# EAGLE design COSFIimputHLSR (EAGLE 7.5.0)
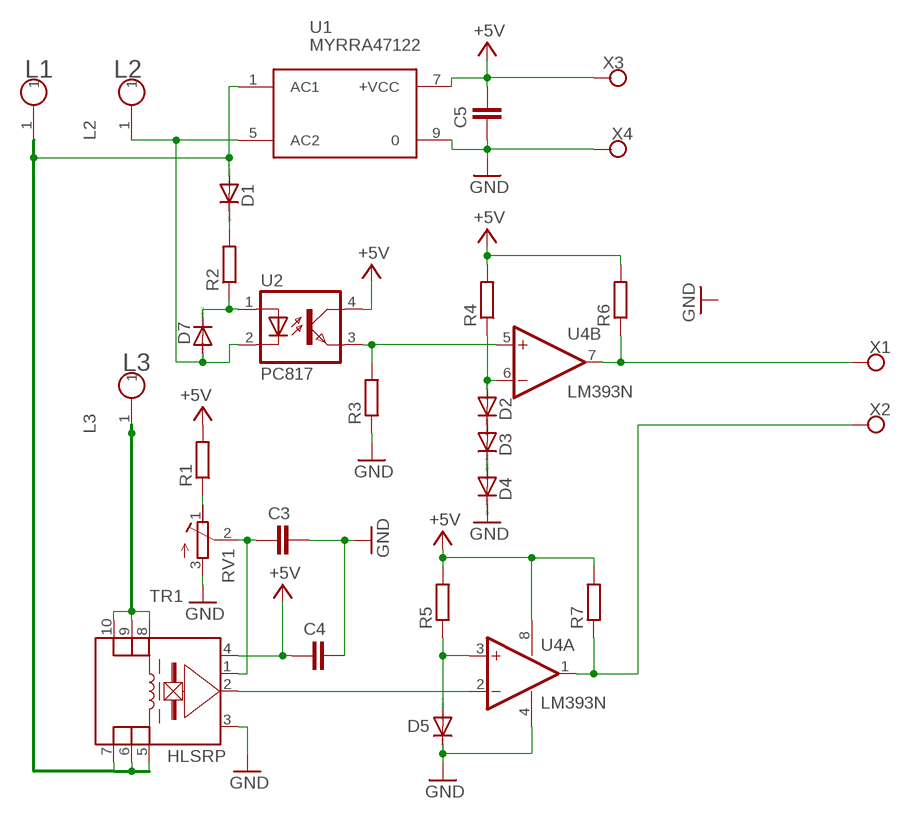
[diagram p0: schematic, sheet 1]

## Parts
C3  C-EUC1206  [C1206]
C4  C-EUC1206  [C1206]
C5  C-EUC1206  [C1206]
D1  1N4004  [DO41-10]
D2  1N4148DO35-7  [DO35-7]
D3  1N4148DO35-7  [DO35-7]
D4  1N4148DO35-7  [DO35-7]
D5  1N4148DO35-7  [DO35-7]
D7  1N4004  [DO41-10]
L1  CONNHOLE  [CONNHOLE4]
L2  CONNHOLE  [CONNHOLE4]
L3  CONNHOLE  [CONNHOLE4]
R1  R-EU_0207/10  [0207/10]
R2  R-EU_0617/22  [0617/22]
R3  R-EU_0204/7  [0204/7]
R4  R-EU_0204/7  [0204/7]
R5  R-EU_0204/7  [0204/7]
R6  R-EU_0204/7  [0204/7]
R7  R-EU_0204/7  [0204/7]
RV1  R-TRIMM-3386-F  [R-TRIMM-3386F]
TR1  HLSRP  [HLRSXPSP]
U1  MYRRA47122  [MYRRA47122]
U2  PC817  [DIL04]
U4  LM393N  [DIL08]
X1  CONNWIRE  [CONNWIRE]
X2  CONNWIRE  [CONNWIRE]
X3  CONNWIRE  [CONNWIRE]
X4  CONNWIRE  [CONNWIRE]

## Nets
+5V: C4.1 C5.2 R1.2 R4.2 R5.2 R6.2 R7.2 TR1.4(V+) U1.7(+VCC) U2.4(COL) U4.8(P:V+) X3.P$1
GND: C3.2 C4.2 C5.1 D4.C D5.C R3.1 RV1.3(E) TR1.3 U1.9 U4.4(P:V-) X4.P$1
N$1: TR1.2 U4.2(A:-IN)
N$2: D5.A R5.1 U4.3(A:+IN)
N$3: D7.C R2.1 U2.1(A)
N$4: D2.C D3.A
N$5: D7.A L2.1 U1.5(AC2) U2.2(C)
N$6: D1.A L1.1 TR1.5(4I-) TR1.6(5I-) TR1.7(6I-) U1.1(AC1)
N$7: C3.1 RV1.2(S) TR1.1
N$8: D3.C D4.A
N$9: R1.1 RV1.1(A)
N$10: D1.C R2.2
N$13: R3.2 U2.3(EMIT) U4.5(B:+IN)
N$16: D2.A R4.1 U4.6(B:-IN)
N$17: R7.1 U4.1(A:OUT) X2.P$1
N$18: R6.1 U4.7(B:OUT) X1.P$1
N$19: L3.1 TR1.8(1I+) TR1.9(2I+) TR1.10(3I+)

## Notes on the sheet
- L1 | L2
- L3

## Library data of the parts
C3-C5 = rcl:C-EU: CAPACITOR, European symbol
D1 D7 = diode:1N4004: DIODE
D2-D5 = diode:1N4148: DIODE
L1-L3 = connholes:CONNHOLE
R1-R7 = rcl:R-EU_: RESISTOR, European symbol
RV1 = rcl:R-TRIMM-3386-F
TR1 = lem:HLSRP
U1 = acdc:MYRRA47122: AC-DC CONVERTER 5V 550mA
U2 = optocoupler:PC817: SHARP OPTO COUPLER; MPN: PC817X4J000F; OC_FARNELL: 9707727; OC_NEWARK: 97K7059
U4 = linear:LM393: COMPARATOR
X1-X4 = connholes:CONNWIRE

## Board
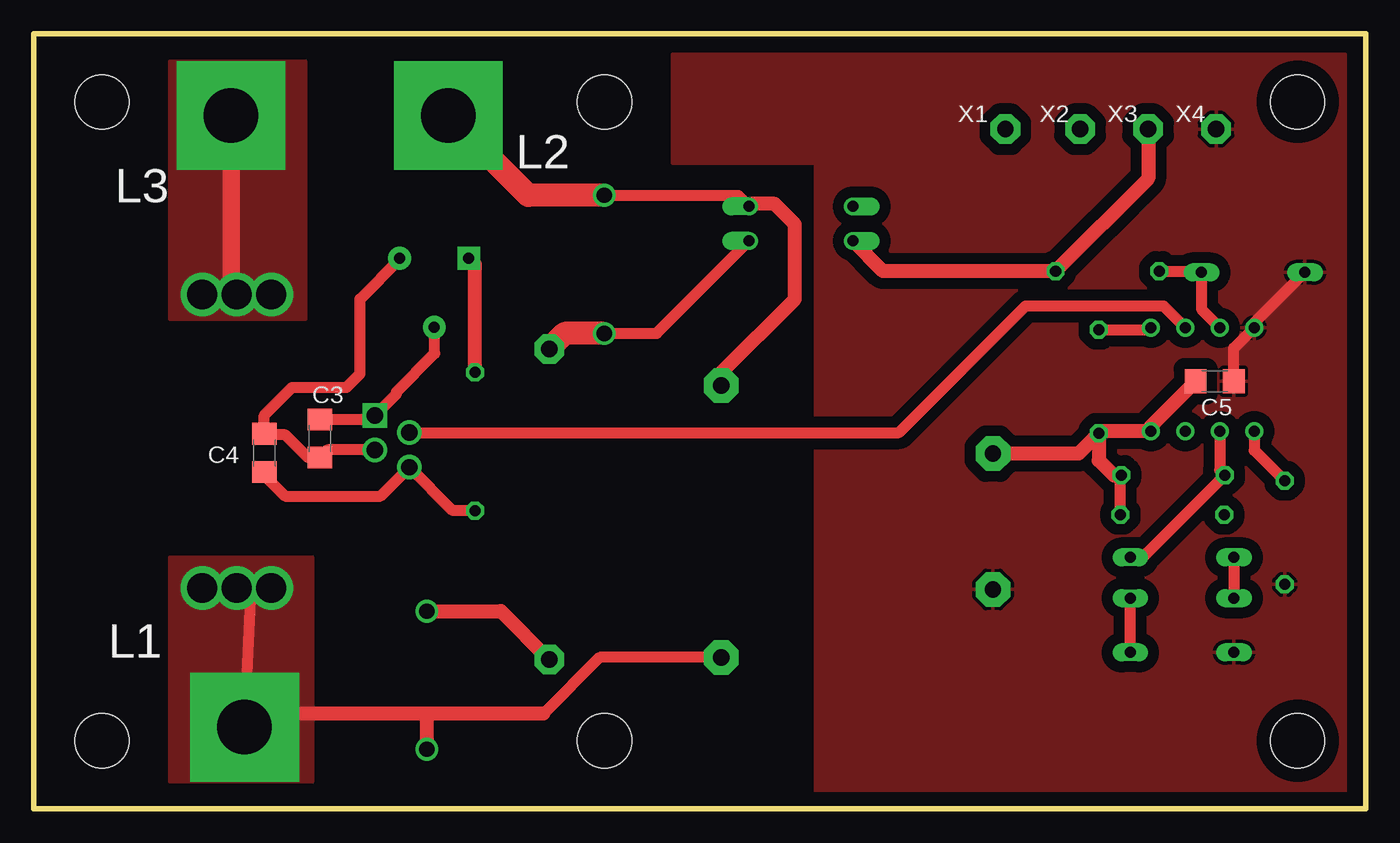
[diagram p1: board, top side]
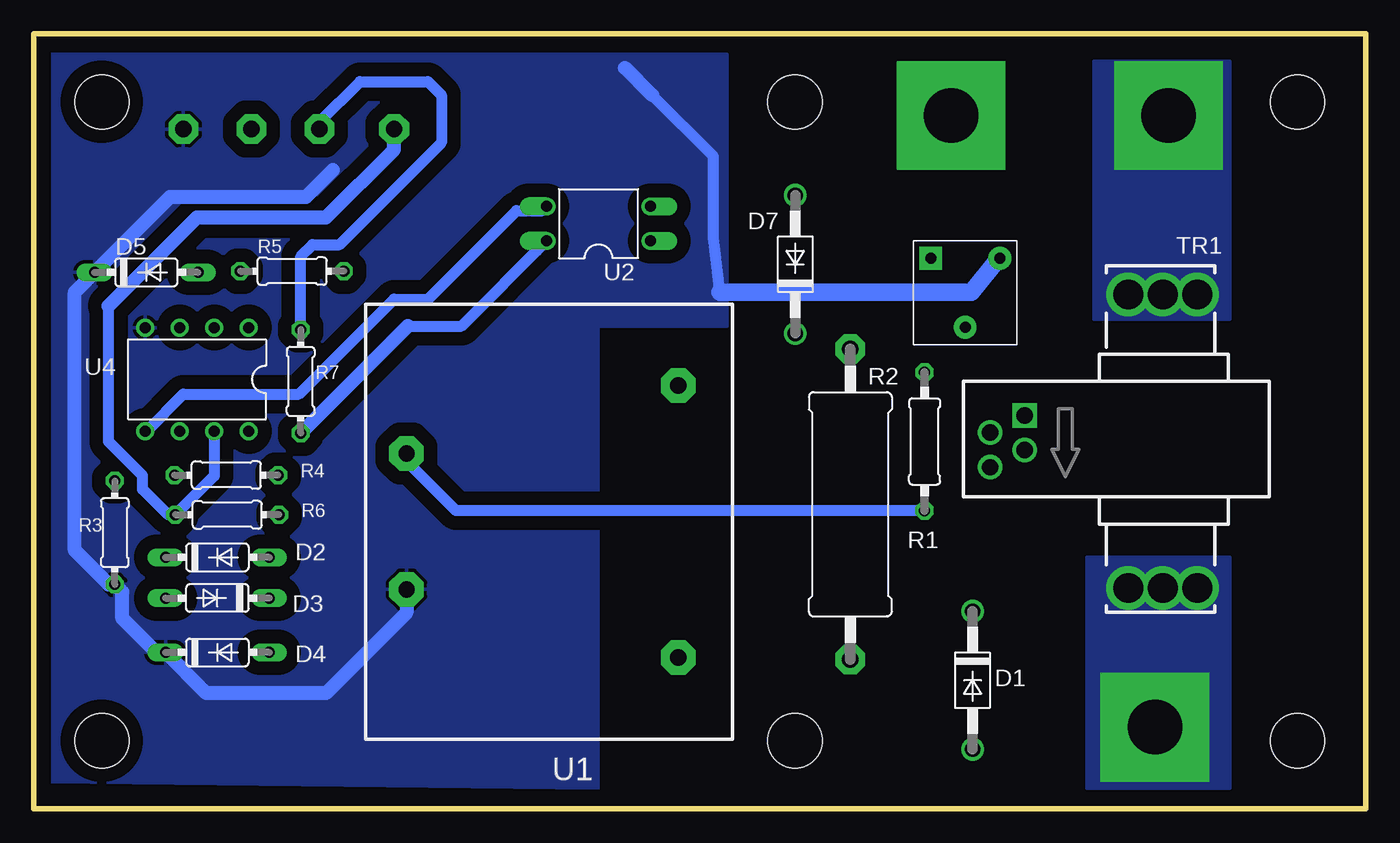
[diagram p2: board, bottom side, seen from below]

Size 98 x 57 mm. Coordinates in mm from the lower left corner, seen from the top.
Outline: 0,0 0,57 98,57 98,0 0,0
Copper layers (1*16): Top 0.035mm / dielectric 1.5mm / Bottom 0.035mm
Design rules "default": minimum track width 10mil, minimum drill 24mil, track to track 8mil, track to pad 8mil, pad to pad 8mil, via to via 8mil, smd to smd 8mil, copper to edge 40mil, drill to drill 8mil, minimum pad ring 10mil, minimum via ring 8mil, stop-mask expansion 4mil, vias tented up to drill 0mil, thermal gap 10mil
Holes 4 mm at 5,5 5,52 93,52 93,5 42,52 42,5

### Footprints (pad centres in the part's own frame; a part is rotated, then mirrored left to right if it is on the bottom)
C1206 = smd 1.6 x 1.8: 1 -1.4,0; 2 1.4,0
DO41-10 = drill 1.118: A 5.08,0; C -5.08,0
DO35-7 = drill 0.813 long: A 3.81,0; C -3.81,0
CONNHOLE4 = drill 4 pad 8 square: 1 0,0
0207/10 = drill 0.813 octagon: 1 -5.08,0; 2 5.08,0
0617/22 = drill 1.2 pad 2.184 octagon: 1 -11.43,0; 2 11.43,0
0204/7 = drill 0.813 octagon: 1 -3.81,0; 2 3.81,0
R-TRIMM-3386F = drill 0.8 pad 1.676 square: 1 0,0 | drill 0.8 pad 1.676: 2 5.08,2.54; 3 0,5.08
HLRSXPSP = drill 1.2 square: 1 0,0 | drill 1.2: 2 1.27,-2.54; 3 2.54,0; 4 3.81,-2.54 | drill 2.2 pad 3.1: 5 12.7,7.62; 6 12.7,10.16; 7 12.7,12.7; 8 -8.89,12.7; 9 -8.89,10.16; 10 -8.89,7.62
MYRRA47122 = drill 1.2 pad 2.54 octagon: 1 0,0; 5 20,0; 7 15,20; 9 5,20
DIL04 = drill 0.813 offset: 1 -1.27,-3.81; 2 1.27,-3.81; 3 1.27,3.81; 4 -1.27,3.81
DIL08 = drill 0.813 pad 1.27: 1 -3.81,-3.81; 2 -1.27,-3.81; 3 1.27,-3.81; 4 3.81,-3.81; 5 3.81,3.81; 6 1.27,3.81; 7 -1.27,3.81; 8 -3.81,3.81
CONNWIRE = drill 1.2 pad 2.184 octagon: P$1 0,0

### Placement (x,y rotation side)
C3  21.05,27.24 270 top
C4  16.95,26.18 90 top
C5  86.9,31.45 180 top
D1  28.92,9.45 270 bottom
D2  84.5,18.5 0 bottom
D3  84.5,15.5 180 bottom
D4  84.5,11.5 0 bottom
D5  89.73,39.47 0 bottom
D7  41.97,40.05 90 bottom
L1  15.5,6 0 top
L2  30.5,51 0 top
L3  14.5,51 0 top
R1  32.45,27.02 270 bottom
R2  37.92,22.4 270 bottom
R3  92.05,20.32 90 bottom
R4  83.84,24.55 0 bottom
R5  79,39.55 0 bottom
R6  83.78,21.63 0 bottom
R7  78.37,31.44 270 bottom
RV1  32,40.5 270 bottom
TR1  25.09,28.94 270 bottom
U1  50.58,11.13 90 bottom
U2  56.45,43.05 90 bottom
U4  86,31.59 180 bottom
X1  71.5,50 0 top
X2  77,50 0 top
X3  82,50 0 top
X4  87,50 0 top

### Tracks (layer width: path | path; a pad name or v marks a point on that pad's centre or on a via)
+5V
  Top 0.813: C4.1 16.95,24.55 18.5,23 25.5,23 TR1.4 30.82,21.94 R1.2 | R6.2 79.97,24.49 R4.2
  Top 1.016: R7.2 78.52,27.78 U4.8 82.19,28.14 C5.2 | R7.2 76.87,26.13 U1.7 | R7.2 78.37,25.63 79.5,24.5 79.98,24.5 R4.2 | U2.4 62.49,39.55 R5.2 82,46.36 X3.P$1
  Bottom 0.813: 61,41.04 U2.4 66.54,35.5 70.5,35.5 | R1.2 66.94,21.94 71,26 70.71,26 U1.7
  Bottom 1.016: 70.5,35.5 R7.2
GND
  Top 0.813: TR1.3 21.61,26.4 C3.2 20.16,25.84 18.5,27.5 17.03,27.5 C4.2 16.95,28.95 19,31 23,31 24,32 24,37.5 26.92,40.42 RV1.3 | C5.1 88.3,33.89 U4.4 89.81,35.74 D5.C
  Bottom 0.813: RV1.3 27,40.5 | 47.5,38 48,42 48,48 52.5,52.5
  Bottom 1.016: U1.9 70.58,14.42 76.5,8.5 85.31,8.5 D4.C 89,11.5 91.5,14 91.5,15.96 R3.1 92.51,16.51 95,19 95,38.01 D5.C 88.01,45 78,45 76,47 | 52.5,52.5 54.5,54.5
  Bottom 1.27: 27,40.5 29,38 47.5,38
  pour Bottom (isolate 1.016): 47,55.5 97,55.5 97,2 56.5,1.5 56.5,35.5 47,35.5
  pour Top (isolate 0.813): 47.5,55.5 96.5,55.5 96.5,2.5 96.5,2 96.5,1 57.5,1 57.5,47.5 47,47.5 47,55.5
N$1
  Top 0.813: TR1.2 63.67,27.67 73,37 83.13,37 U4.2
N$2
  Top 0.813: R5.1 85.84,39.55 D5.A 85.92,36.75 U4.3
N$3
  Top 0.813: D7.C 45.83,34.97 U2.1
  Top 1.676: D7.C 39.06,34.97 R2.1
N$4
  Top 0.813: D2.C D3.A
N$5
  Top 0.813: D7.A 51.83,45.13 U2.2
  Top 1.016: U1.5 50.58,32.08 56,37.5 56,43 54.5,44.5 52.82,44.5 U2.2
  Top 1.676: D7.A 36.37,45.13 L2.1
N$6
  Top 0.813: TR1.7 TR1.6 16,16.24 | TR1.5 16,16.24 | L1.1 16,16.24 | U1.1 41.63,11.13 37.5,7
  Top 1.016: 37.5,7 29,7 | 29,7 17.5,7 16.5,6 L1.1 | D1.A 28.92,6.92 29,7
  pour Top (no thermals): 10,18.5 20.5,18.5 20.5,2 10,2
  pour Bottom (no thermals): 10,18.5 20.5,18.5 20.5,1.5 10,1.5 10,2.5
N$7
  Top 0.813: C3.1 24.79,28.64 TR1.1 26.66,30.51 26.66,30.66 29.5,33.5 29.5,35.38 RV1.2
N$8
  Top 0.813: D4.A D3.C
N$9
  Top 1.016: R1.1 32.45,40.05 RV1.1
N$10
  Top 1.016: D1.C 34.36,14.53 R2.2
N$13
  Top 0.813: U4.5 89.81,26.37 R3.2
  Bottom 0.813: U4.5 89.72,27.78 87,30.5 78.5,30.5 71.5,37.5 69,37.5 62.5,44 60.58,44 U2.3
N$16
  Top 0.813: U4.6 87.27,24.93 R4.1 81.6,18.5 D2.A
N$17
  Top 0.813: R7.1 82.04,35.25 U4.1
  Bottom 0.813: R7.1 78.37,40.63 77.5,41.5 75.5,41.5 68,49 68,52.5 69,53.5 74,53.5 77,50.5 X2.P$1
N$18
  Bottom 0.813: 92.5,37 92.5,27 90,24.5 90,23.5 88.13,21.63 R6.1 84.73,24.49 U4.7
  Bottom 1.016: 92.5,37 86,43.5 76.5,43.5 71.5,48.5 X1.P$1
N$19
  Top 1.27: L3.1 14.5,38.26 TR1.9 | TR1.8 14,37.83 TR1.9 | TR1.10 TR1.9
  pour Top (no thermals): 10,55 20,55 20,36 10,36
  pour Bottom (no thermals): 10,55 20,55 20,36 10,36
